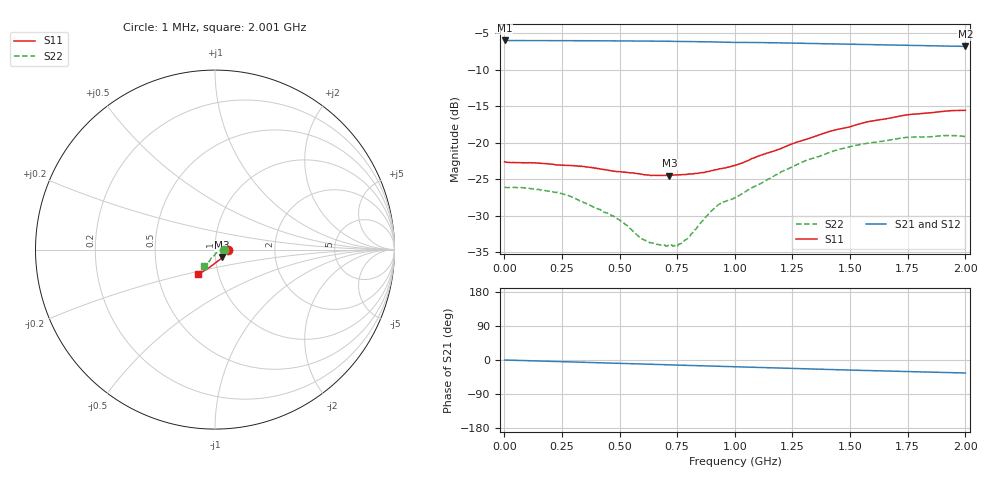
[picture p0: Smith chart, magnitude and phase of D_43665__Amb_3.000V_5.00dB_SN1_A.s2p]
! device id: 43665_
! dir: \\malibu\benchdata\1_engineers\tn_data\43665_75ohm\new\sparar\43665_\amb\3p000v\5p00db
! Serial: 1
! Insertion: A
! Temp: Amb
! VDD: 3.000V
! Attenuation Step: 5.00dB
! IDD: 1.452945e+00mA
! FILE NAME
! DATE 03-27-2009 08:34:36
! CORRECTED  DATA
#  Hz  S  RI  R  75
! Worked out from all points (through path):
!   401 points, 1 MHz to 2.001 GHz, reference 75 ohm
!   highest |S21| = -5.98 dB at 1 MHz (marker M1); lowest = -6.8 dB at 2.001 GHz (marker M2)
!   group delay of S21, straight-line fit = 48.5 ps
!   lowest |S11| = -24.5 dB at 716 MHz (marker M3), VSWR 1.13, Z = 81 - j7.13 ohm
!   |S11| at or under -10 dB: start of sweep to end of sweep
!   |S22| runs from -34.2 to -19.0 dB; largest |S21 - S12| = 0.0022
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1000000  0.0741 -0.0013  0.5024 -0.000687  0.5023 -0.000848  0.0499 -0.000777
9.6e7  0.0726 -0.00423  0.5013 -0.0146  0.5015 -0.0147  0.0489 0.00116
2.31e8  0.0695 -0.0106  0.4998 -0.0352  0.5 -0.0353  0.0457 0.00144
3.36e8  0.0671 -0.0165  0.4978 -0.0513  0.4979 -0.0514  0.0395 0.0016
4.81e8  0.0587 -0.0249  0.4938 -0.0736  0.4939 -0.0738  0.0305 -0.00315
6.06e8  0.0496 -0.0344  0.4888 -0.0924  0.4887 -0.0926  0.0199 -0.00831
6.71e8  0.0441 -0.04  0.4861 -0.1025  0.486 -0.1026  0.0155 -0.0126
7.16e8  0.0402 -0.0439  0.4839 -0.1095  0.4839 -0.1096  0.0122 -0.0154
7.41e8  0.0381 -0.0465  0.4826 -0.1134  0.4826 -0.1135  0.0102 -0.0168
7.71e8  0.0351 -0.0491  0.4808 -0.1181  0.4808 -0.1181  0.0071 -0.0192
8.01e8  0.0321 -0.0519  0.479 -0.1228  0.4789 -0.1228  0.00401 -0.0222
8.76e8  0.0229 -0.0588  0.4734 -0.1345  0.4735 -0.1344  -0.00205 -0.0311
9.21e8  0.0168 -0.0632  0.4689 -0.1407  0.4691 -0.1405  -0.0075 -0.0358
9.46e8  0.0143 -0.065  0.4666 -0.1432  0.4668 -0.143  -0.012 -0.0369
1.001e9  0.00866 -0.0694  0.464 -0.149  0.4643 -0.1489  -0.0175 -0.038
1.211e9  -0.0197 -0.0906  0.4492 -0.1784  0.4497 -0.1786  -0.0272 -0.0581
1.336e9  -0.0362 -0.1026  0.438 -0.1934  0.4387 -0.1937  -0.0349 -0.0696
1.491e9  -0.0557 -0.1148  0.4235 -0.211  0.4239 -0.2118  -0.0437 -0.0821
1.671e9  -0.0755 -0.1266  0.4072 -0.2293  0.407 -0.2304  -0.0515 -0.0906
1.751e9  -0.0828 -0.1316  0.3998 -0.2367  0.3997 -0.2382  -0.0547 -0.0942
1.901e9  -0.0927 -0.1348  0.3863 -0.2495  0.3855 -0.2497  -0.0617 -0.0933
2.001e9  -0.0965 -0.1359  0.3779 -0.2574  0.3761 -0.2587  -0.0632 -0.0901
